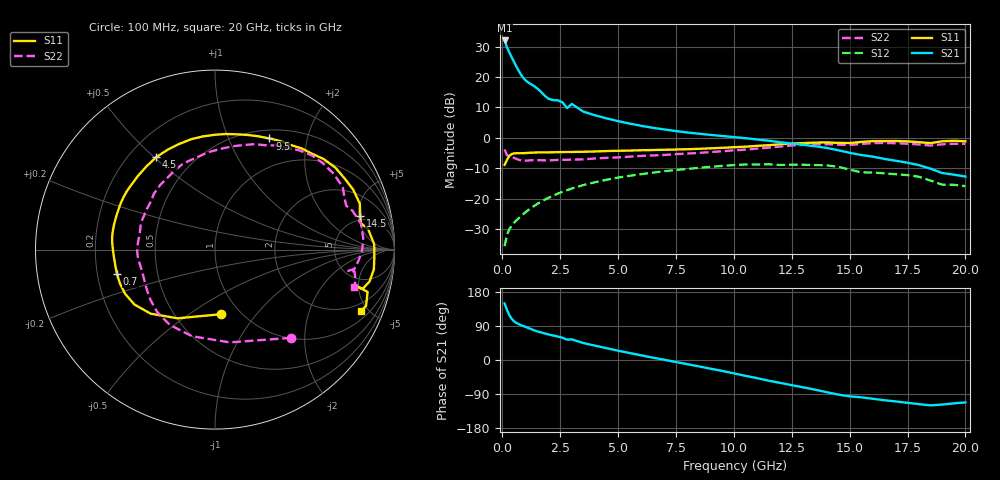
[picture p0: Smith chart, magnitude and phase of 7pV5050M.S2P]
! Infineon Technologies  Discrete & RF Semiconductors
! bfp620
! VCE = 0.50 V,  IC =  50 mA
! Common Emitter S-Parameters:  Sep 2002
# GHz  S  MA  R  50
!  f  S11  S21  S12  S22
! GHz  MAG  ANG  MAG  ANG  MAG  ANG  MAG  ANG
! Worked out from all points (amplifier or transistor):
!   59 points, 100 MHz to 20 GHz, reference 50 ohm
!   highest |S21| = 32.0 dB at 100 MHz (marker M1)
!   |S21| within 3 dB of that: start of sweep to 246.9 MHz
!   unconditionally stable (mu >= 1): 1.785 GHz to 10.65 GHz; 16.85 GHz to end of sweep
!   at 1 GHz: K = 0.92, MSG = 21.7 dB, |S12| = -24.4 dB
!   at 5.5 GHz: K = 1.07, MAG = 7.0 dB, |S12| = -12.4 dB
!   at 20 GHz: K = 1.76, MAG = -3.5 dB, |S12| = -15.8 dB
!   S11 on the Smith chart (normalised r, x): 100 MHz: 0.81, -0.67; 700 MHz: 0.28, -0.11; 4.5 GHz: 0.31, +0.51; 9.5 GHz: 0.60, +1.43; 14.5 GHz: 4.39, +5.24; 20 GHz: 1.45, -4.49
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0.1  0.3615 -85.0  39.77 149.2  0.0168 50.2  0.6486 -49.3
0.2  0.436 -118.6  30.85 132.3  0.0254 47.4  0.5235 -81.0
0.3  0.5059 -135.1  25.39 118.8  0.0316 46.9  0.4993 -104.9
0.4  0.5432 -145.7  21.33 109.2  0.0363 47.3  0.4893 -121.0
0.5  0.5583 -153.8  17.94 102.6  0.0404 48.0  0.4739 -132.8
0.6  0.5623 -160.4  15.08 98.0  0.0442 48.9  0.4558 -142.1
0.7  0.5624 -166.0  12.78 94.8  0.048 49.8  0.4402 -149.8
0.8  0.5624 -170.6  11.01 92.2  0.052 50.6  0.4297 -156.1
1  0.566 -177.5  8.858 87.5  0.0603 51.8  0.4242 -165.3
1.4  0.577 173.1  6.988 77.9  0.078 52.2  0.4331 -176.6
1.9  0.58 162.0  4.69 69.0  0.1 50.1  0.429 170.0
2.8  0.5892 146.6  3.091 53.7  0.1393 43.1  0.4388 153.3
3  0.589 144.4  3.619 54.5  0.1482 41.2  0.4413 152.5
3.5  0.5938 136.5  2.702 44.7  0.1688 36.2  0.4455 144.2
4.5  0.6104 122.4  2.099 31.3  0.2062 26.2  0.4725 130.1
7  0.6399 90.0  1.378 0.6  0.2851 0.2  0.5266 99.7
9.5  0.6897 63.9  1.077 -28.9  0.3482 -26.9  0.6055 74.3
10.5  0.7195 54.1  0.992 -41.7  0.367 -39.6  0.6437 64.7
13.5  0.8394 23.4  0.731 -78.2  0.3596 -74.8  0.7846 32.6
14.5  0.8303 12.9  0.63 -91.2  0.3373 -90.2  0.7757 21.3
17  0.8919 -7.1  0.423 -109.4  0.2542 -105.7  0.8204 -0.1
20  0.882 -22.9  0.233 -111.9  0.1623 -117.3  0.801 -14.9
